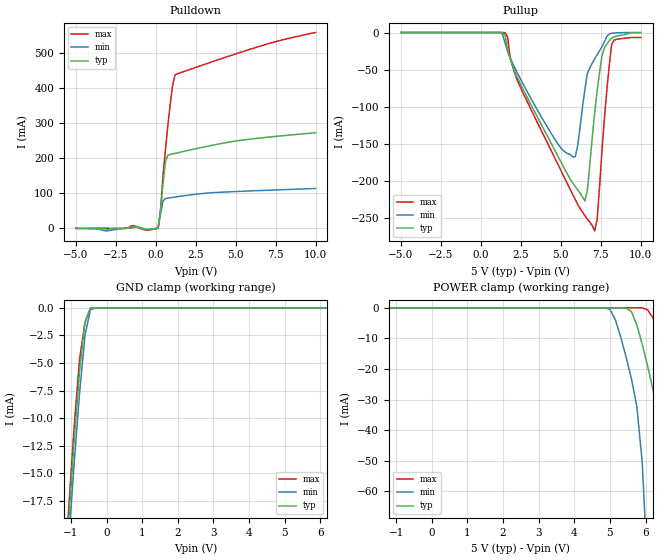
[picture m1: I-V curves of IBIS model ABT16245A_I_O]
|   TEXAS INSTRUMENTS INCORPORATED
|   Advanced Bus Interface Group
|   IBIS Model of SN74ABT16245A
|   16-BIT BUS TRANSCEIVERS WITH 3-STATE OUTPUTS
|   48-pin DGG,DL Package
[IBIS Ver]   2.1
[Comment char]  |_char
[File Name]   abt16245a.ibs
[File Rev]   1.0
[Date]   7/22/98
[Source]   File originated at Texas Instruments Incorporated.
[Notes]   The following is a sample IBIS file for the ABT16245a.
   - This file may be incomplete or may not be fully compliant
   with the IBIS specification. It will be replaced with a
   version that is IBIS Revision 3.2 compliant and is complete
   and accurate. Please email all questions and comments to
   sllibis@ti.com.
|   - All test data contained in this file are derived from
|   hspice(tm) simulations.
|   - File created by Ramzi Ammar, SLL Applications
[Disclaimer] Property of Texas Instruments Incorporated.  Unauthorized
   reproduction and/or distribution is strictly prohibited.
   This product is protected under copyright law.
   Created 1998, (C) Copyright 1998, Texas Instruments
   Incorporated, All Rights Reserved
   UNLESS THERE IS A SIGNED, WRITTEN AGREEMENT TO THE
   CONTRARY, TEXAS INSTRUMENTS ("TI") IS PROVIDING THE IBIS
   MODELS "AS IS" AND WITHOUT ANY WARRANTY, EXPRESSED OR
   IMPLIED.  TI assumes no liability for:
   1) the accuracy of the IBIS models provided to your
   company;
   2) the proper functioning of these IBIS models in your
   design or for any resulting applications; or
   3) infringement of patents, copyrights or intellectual
   property rights resulting from your use of these IBIS
   models.
   TI provides IBIS Models as a service to our customers.
   You and your company shall not distribute, sell or give
   these models to anyone else without prior written
   permission from TI.
   TI reserves the right to make changes to our products or
   to discontinue any semiconductor product or service
   without notice, and advises our customers to obtain the
   latest version of relevant information to verify, before
   placing orders, that the information being relied on is
   current.
   Please be aware that your receipt and use of the IBIS
   information provided shall serve as acceptance of these
   terms and conditions.  If you do not accept these terms,
   you should return or destroy the IBIS models and any
   other accompanying information immediately.
|   TSSOP   PACKAGE   (DGG)
[Component]   ABT16245A_DGG
[manufacturer]   Texas Instruments Incorporated
[Package]
|   typ   min   max
R_pkg   0.044   0.038   0.051
L_pkg   3.019nH   2.486nH   4.099nH
C_pkg   0.507pF   0.334pF   0.809pF
[Pin]   signal_name   model_name   R_pin   L_pin   C_pin
1   1DIR   NC   0.041   4.017nH   0.759pF
2   1B1   ABT16245A_I_O   0.042   3.737nH   0.792pF
3   1B2   ABT16245A_I_O   0.042   3.48nH   0.661pF
4   GND   GND   0.038   3.131nH   0.575pF
5   1B3   ABT16245A_I_O   0.047   3.122nH   0.566pF
6   1B4   ABT16245A_I_O   0.043   2.948nH   0.504pF
7   VCC   POWER   0.045   2.845nH   0.397pF
8   1B5   ABT16245A_I_O   0.049   2.835nH   0.394pF
9   1B6   ABT16245A_I_O   0.048   2.715nH   0.378pF
10   GND   GND   0.05   2.664nH   0.363pF
11   1B7   ABT16245A_I_O   0.05   2.585nH   0.348pF
12   1B8   ABT16245A_I_O   0.049   2.55nH   0.337pF
13   2B1   ABT16245A_I_O   0.049   2.541nH   0.336pF
14   2B2   ABT16245A_I_O   0.05   2.574nH   0.348pF
15   GND   GND   0.049   2.618nH   0.359pF
16   2B3   ABT16245A_I_O   0.046   2.671nH   0.375pF
17   2B4   ABT16245A_I_O   0.045   2.754nH   0.389pF
18   VCC   POWER   0.044   2.823nH   0.45pF
19   2B5   ABT16245A_I_O   0.042   2.968nH   0.503pF
20   2B6   ABT16245A_I_O   0.051   3.108nH   0.535pF
21   GND   GND   0.042   3.175nH   0.587pF
22   2B7   ABT16245A_I_O   0.041   3.449nH   0.678pF
23   2B8   ABT16245A_I_O   0.044   3.766nH   0.804pF
24   2DIR   NC   0.043   4.065nH   0.761pF
25   2OE_BAR   NC   0.041   3.994nH   0.757pF
26   2A8   ABT16245A_I_O   0.039   3.649nH   0.789pF
27   2A7   ABT16245A_I_O   0.038   3.362nH   0.66pF
28   GND   GND   0.038   3.082nH   0.574pF
29   2A6   ABT16245A_I_O   0.044   2.99nH   0.522pF
30   2A5   ABT16245A_I_O   0.041   2.917nH   0.495pF
31   VCC   POWER   0.043   2.82nH   0.448pF
32   2A4   ABT16245A_I_O   0.043   2.699nH   0.385pF
33   2A3   ABT16245A_I_O   0.045   2.628nH   0.372pF
34   GND   GND   0.046   2.556nH   0.356pF
35   2A2   ABT16245A_I_O   0.046   2.495nH   0.344pF
36   2A1   ABT16245A_I_O   0.047   2.487nH   0.334pF
37   1A8   ABT16245A_I_O   0.047   2.49nH   0.335pF
38   1A7   ABT16245A_I_O   0.046   2.486nH   0.343pF
39   GND   GND   0.045   2.566nH   0.356pF
40   1A6   ABT16245A_I_O   0.044   2.639nH   0.374pF
41   1A5   ABT16245A_I_O   0.043   2.701nH   0.386pF
42   VCC   POWER   0.043   2.817nH   0.45pF
43   1A4   ABT16245A_I_O   0.041   2.935nH   0.501pF
44   1A3   ABT16245A_I_O   0.047   3.035nH   0.529pF
45   GND   GND   0.043   3.171nH   0.589pF
46   1A2   ABT16245A_I_O   0.04   3.415nH   0.682pF
47   1A1   ABT16245A_I_O   0.043   3.741nH   0.809pF
48   1OE_BAR   NC   0.044   4.099nH   0.764pF
|   SSOP   PACKAGE   (DL)
[Component]   ABT16245A_DL
[manufacturer]   Texas Instruments Incorporated
[Package]
|   typ   min   max
R_pkg   0.048   0.038   0.053
L_pkg   6.046nH   5.084nH   7.968nH
C_pkg   0.813pF   0.569pF   1.157pF
[Pin]   signal_name   model_name   R_pin   L_pin   C_pin
1   1DIR   NC   0.046   7.968nH   1.017pF
2   1B1   ABT16245A_I_O   0.044   7.299nH   1.157pF
3   1B2   ABT16245A_I_O   0.043   6.765nH   1.058pF
4   GND   GND   0.041   6.269nH   0.933pF
5   1B3   ABT16245A_I_O   0.038   5.856nH   0.829pF
6   1B4   ABT16245A_I_O   0.046   5.802nH   0.79pF
7   VCC   POWER   0.05   5.656nH   0.738pF
8   1B5   ABT16245A_I_O   0.053   5.5nH   0.643pF
9   1B6   ABT16245A_I_O   0.052   5.304nH   0.606pF
10   GND   GND   0.053   5.189nH   0.583pF
11   1B7   ABT16245A_I_O   0.051   5.084nH   0.569pF
12   1B8   ABT16245A_I_O   0.053   5.862nH   0.833pF
13   2B1   ABT16245A_I_O   0.053   5.862nH   0.833pF
14   2B2   ABT16245A_I_O   0.051   5.084nH   0.569pF
15   GND   GND   0.053   5.189nH   0.583pF
16   2B3   ABT16245A_I_O   0.052   5.304nH   0.606pF
17   2B4   ABT16245A_I_O   0.053   5.5nH   0.643pF
18   VCC   POWER   0.05   5.656nH   0.738pF
19   2B5   ABT16245A_I_O   0.046   5.802nH   0.79pF
20   2B6   ABT16245A_I_O   0.038   5.856nH   0.829pF
21   GND   GND   0.041   6.269nH   0.933pF
22   2B7   ABT16245A_I_O   0.043   6.765nH   1.058pF
23   2B8   ABT16245A_I_O   0.044   7.299nH   1.157pF
24   2DIR   NC   0.046   7.968nH   1.017pF
25   2OE_BAR   NC   0.046   7.968nH   1.017pF
26   2A8   ABT16245A_I_O   0.044   7.299nH   1.157pF
27   2A7   ABT16245A_I_O   0.043   6.765nH   1.058pF
28   GND   GND   0.041   6.269nH   0.933pF
29   2A6   ABT16245A_I_O   0.038   5.856nH   0.829pF
30   2A5   ABT16245A_I_O   0.046   5.802nH   0.79pF
31   VCC   POWER   0.05   5.656nH   0.738pF
32   2A4   ABT16245A_I_O   0.053   5.5nH   0.643pF
33   2A3   ABT16245A_I_O   0.052   5.304nH   0.606pF
34   GND   GND   0.053   5.189nH   0.583pF
35   2A2   ABT16245A_I_O   0.051   5.084nH   0.569pF
36   2A1   ABT16245A_I_O   0.053   5.862nH   0.833pF
37   1A8   ABT16245A_I_O   0.053   5.862nH   0.833pF
38   1A7   ABT16245A_I_O   0.051   5.084nH   0.569pF
39   GND   GND   0.053   5.189nH   0.583pF
40   1A6   ABT16245A_I_O   0.052   5.304nH   0.606pF
41   1A5   ABT16245A_I_O   0.053   5.5nH   0.643pF
42   VCC   POWER   0.05   5.656nH   0.738pF
43   1A4   ABT16245A_I_O   0.046   5.802nH   0.79pF
44   1A3   ABT16245A_I_O   0.038   5.856nH   0.829pF
45   GND   GND   0.041   6.269nH   0.933pF
46   1A2   ABT16245A_I_O   0.043   6.765nH   1.058pF
47   1A1   ABT16245A_I_O   0.044   7.299nH   1.157pF
48   1OE_BAR   NC   0.046   7.967nH   1.017pF
| Models and submodels in the file (1): ABT16245A_I_O (I/O)
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|   Model ABT16245A_IO
[Model]   ABT16245A_I_O
Model_type   I/O
Polarity   Inverting
Enable   Active-Low
Vinl = 0.8V
Vinh = 2.0V
|   typ   min   max
C_comp   7pF   NA   NA
[Temperature Range]   25   -40   85
[Voltage range]   5.0   4.5   5.5
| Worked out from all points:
|   slope of the pulldown table from 0 to 0.75 V, typ, clamps not added: 3.59 ohm
|   GND clamp passes 1 mA (typ) near -0.57 V on its own axis
[Pullup]   | Vtable = Vcc - Voutput
|   Voltage   I(typ)   I(min)   I(max)
-5V       -522.3pA   -416.2pA   -588pA
1.514V    -3.877mA   -14.55mA   -293.1uA
2.272V    -60.44mA   -54.21mA   -64.06mA
5.756V    -203.6mA   -168.3mA   -219.4mA
6.059V    -212.9mA   -152.5mA   -232.4mA
6.514V    -227.6mA   -75.56mA   -247.6mA
6.665V    -212.2mA   -54.97mA   -252.2mA
7.12V     -108.6mA   -35.64mA   -268mA
7.271V    -79.54mA   -30.05mA   -253.2mA
7.574V    -31.7mA    -19.19mA   -160.3mA
8.181V    -7.744mA   -1.067mA   -16.27mA
9.998V    -471.6uA   -23.7uA    -6.796mA
[pulldown]
|   Voltage   I(typ)   I(min)   I(max)
-5V       -46.5uA    -186.8uA   -700uA
-3.03V    -3.087mA   -7.618mA   -197.4uA
-1.364V   4.369mA    1.615mA    7.242mA
151mV     587.3uA    1.825mA    -483.4uA
302.5mV   50.73mA    39.98mA    50.75mA
454mV     127.1mA    77.48mA    149.7mA
605.5mV   188.9mA    84.77mA    223.2mA
757mV     208.8mA    85.95mA    292mA
1.06V     212.3mA    88.08mA    410mA
1.212V    213.9mA    89.11mA    438.4mA
5.151V    250.1mA    105.1mA    500.5mA
9.998V    273mA      113.5mA    559.4mA
[gnd_clamp]
|   Voltage   I(typ)   I(min)   I(max)
-5V       -993.1mA   -927.1mA   -1.042A
-1.212V   -26.97mA   -29.2mA    -26.17mA
-1.061V   -19.16mA   -21.09mA   -18.05mA
-909.5mV  -12.04mA   -14.09mA   -10.75mA
-758mV    -5.705mA   -7.731mA   -4.667mA
-606.5mV  -1.285mA   -2.506mA   -1.346mA
-455mV    -52.93uA   -193.3uA   -42.81uA
-303.5mV  -327.8nA   -2.555uA   -56.65nA
9.998V    8.635nA    9.207nA    8.613nA
[power_clamp]   | Vtable = Vcc - Voutput
|   Voltage   I(typ)   I(min)   I(max)
-5V       8.637nA    8.751nA    9.051nA
4.999V    -1.597nA   -498.4uA   209.2pA
5.302V    -313.1nA   -9.495mA   -60.06pA
5.605V    -1.26mA    -23.26mA   -2.165nA
5.756V    -5.647mA   -32.32mA   -14.21nA
5.908V    -11.97mA   -50.79mA   -1.882uA
6.059V    -19.08mA   -87.06mA   -665.9uA
6.362V    -35.65mA   -186mA     -8.655mA
6.665V    -92.25mA   -280.5mA   -23.55mA
6.968V    -218.1mA   -344.9mA   -41.82mA
7.271V    -338.4mA   -408.4mA   -96.36mA
9.998V    -992.8mA   -1.04A     -925.7mA
[ramp]
| variable   typ   min   max
dV/dt_r   1.6840E+00/9.2223E-10  1.4308E+00/1.3684E-09  1.9190E+00/6.3113E-10
dV/dt_f   2.7718E+00/5.9758E-10  2.4156E+00/9.7171E-10  3.0786E+00/5.2514E-10
